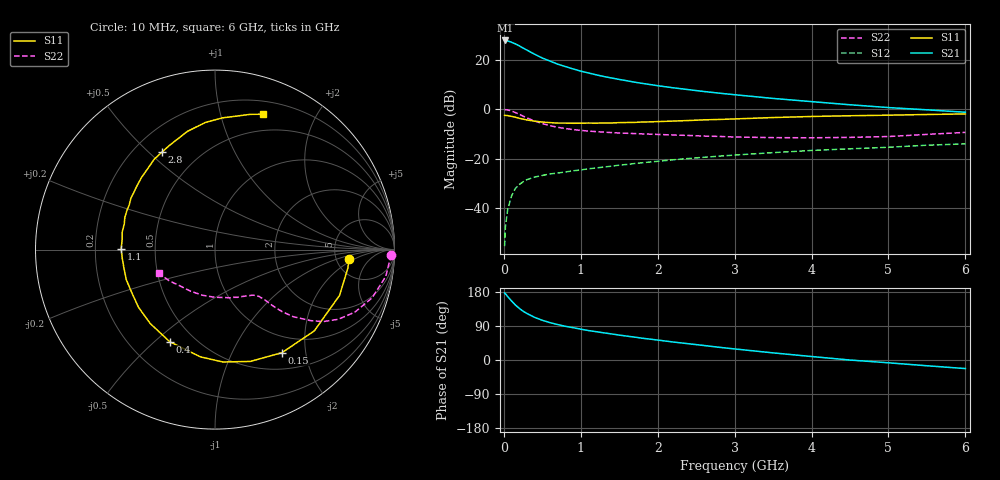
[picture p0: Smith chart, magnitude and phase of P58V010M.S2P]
! SIEMENS Small Signal Semiconductors
! BFP183
! Si NPN RF Bipolar Junction Transistor in SOT143
! VCE = 8 V  IC = 10 mA
! Common Emitter S-Parameters:  March  1996
# GHz  S  MA  R  50
!  f  S11  S21  S12  S22
! GHz  MAG  ANG  MAG  ANG  MAG  ANG  MAG  ANG
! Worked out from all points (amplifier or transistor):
!   36 points, 10 MHz to 6 GHz, reference 50 ohm
!   highest |S21| = 27.8 dB at 20 MHz (marker M1)
!   |S21| within 3 dB of that: start of sweep to 246.1 MHz
!   unconditionally stable (mu >= 1): 1.264 GHz to 5.661 GHz
!   at 250 MHz: K = 0.30, MSG = 27.0 dB, |S12| = -29.4 dB
!   at 1.4 GHz: K = 1.05, MAG = 16.5 dB, |S12| = -23.1 dB
!   at 6 GHz: K = 0.97, MSG = 6.4 dB, |S12| = -14.0 dB
!   lowest NFmin = 1.30 dB at 450 MHz
!   S11 on the Smith chart (normalised r, x): 10 MHz: 6.63, -1.54; 150 MHz: 0.73, -1.59; 400 MHz: 0.37, -0.56; 1.1 GHz: 0.31, +0.00; 2.8 GHz: 0.31, +0.55; 6 GHz: 0.33, +1.36
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0.01  0.7498 -3.9  24.31 177.1  0.0017 79.4  0.9832 -1.7
0.02  0.7471 -8.1  24.42 175.0  0.0041 86.8  0.9751 -3.6
0.05  0.7393 -20.2  23.87 167.3  0.0094 81.4  0.9634 -8.9
0.1  0.715 -39.3  22.45 155.9  0.0176 70.3  0.9155 -17.1
0.15  0.6849 -57.0  20.81 145.2  0.025 63.4  0.8535 -24.1
0.2  0.6533 -72.5  19.02 136.4  0.0299 57.9  0.7885 -29.5
0.25  0.6277 -86.0  17.15 128.8  0.034 53.5  0.7233 -33.7
0.3  0.6031 -97.7  15.61 122.7  0.0376 50.1  0.6637 -36.6
0.4  0.5718 -116.2  12.86 112.5  0.0423 45.8  0.5747 -40.6
0.5  0.5475 -131.3  10.78 104.8  0.0457 42.8  0.511 -42.7
0.6  0.5339 -143.0  9.354 98.6  0.049 41.5  0.4633 -43.9
0.7  0.5221 -152.4  8.109 93.5  0.0511 41.6  0.4289 -44.6
0.8  0.5218 -161.2  7.249 88.9  0.0537 41.0  0.4051 -45.0
1.1  0.5225 179.4  5.377 77.7  0.0623 41.4  0.3594 -46.7
1.3  0.5261 169.4  4.562 71.7  0.0676 42.1  0.3428 -48.5
1.6  0.5367 156.1  3.741 63.0  0.0762 42.4  0.3249 -51.6
2.2  0.5736 135.6  2.7 47.5  0.0946 40.9  0.2998 -60.9
2.8  0.6183 118.6  2.102 33.5  0.1122 37.8  0.2808 -73.2
3.5  0.6761 103.2  1.646 18.8  0.1321 33.7  0.2655 -90.5
4.5  0.735 86.8  1.225 -0.1  0.1578 26.5  0.2685 -119.9
5.5  0.7787 75.4  0.968 -15.2  0.1866 20.1  0.3085 -145.7
6  0.7996 70.6  0.864 -22.6  0.1986 16.0  0.3389 -157.1
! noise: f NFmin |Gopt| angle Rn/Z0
0.45  1.3  0.15  45  0.18
0.9  1.4  0.2  125  0.19
1.8  2.1  0.34  -170  0.14
